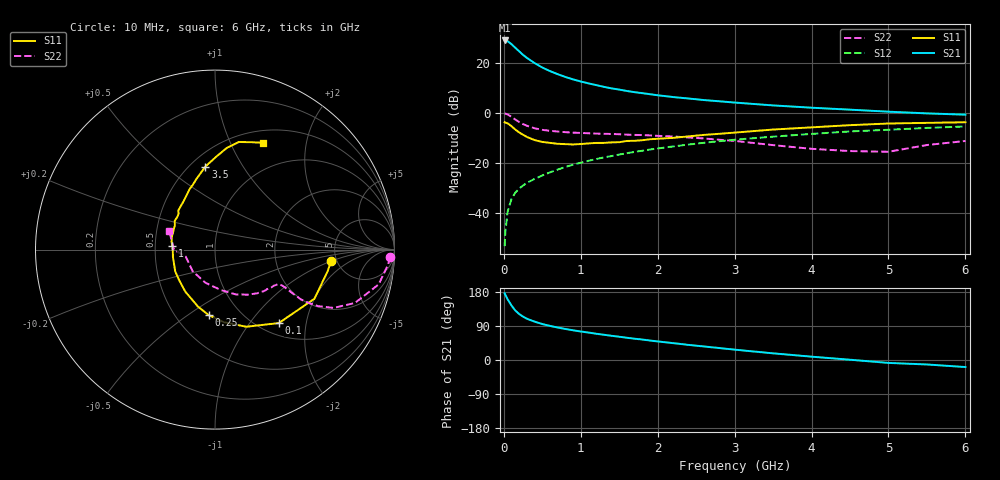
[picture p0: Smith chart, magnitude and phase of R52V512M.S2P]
! SIEMENS Small Signal Semiconductors
! BFR183
! Si NPN RF Bipolar Junction Transistor in SOT23
! VCE = 2.5 V  IC = 12 mA
! Common Emitter S-Parameters:  May  1996
# GHz  S  MA  R  50
!  f  S11  S21  S12  S22
! GHz  MAG  ANG  MAG  ANG  MAG  ANG  MAG  ANG
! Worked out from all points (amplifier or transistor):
!   36 points, 10 MHz to 6 GHz, reference 50 ohm
!   highest |S21| = 28.9 dB at 10 MHz (marker M1)
!   |S21| within 3 dB of that: start of sweep to 151.7 MHz
!   unconditionally stable (mu >= 1): 696 MHz to 2.461 GHz
!   at 250 MHz: K = 0.68, MSG = 26.1 dB, |S12| = -29.0 dB
!   at 1.4 GHz: K = 1.06, MAG = 12.1 dB, |S12| = -17.2 dB
!   at 6 GHz: K = 0.90, MSG = 2.3 dB, |S12| = -5.4 dB
!   S11 on the Smith chart (normalised r, x): 10 MHz: 4.49, -0.95; 100 MHz: 1.21, -1.41; 250 MHz: 0.72, -0.60; 1 GHz: 0.61, +0.03; 3.5 GHz: 0.59, +0.70; 6 GHz: 0.64, +1.33
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0.01  0.6494 -5.4  27.82 175.9  0.0022 84.9  0.9757 -2.4
0.02  0.6392 -10.9  27.72 171.6  0.0043 85.0  0.9686 -4.9
0.05  0.6178 -26.3  26.83 160.0  0.0109 80.0  0.9322 -12.0
0.1  0.5423 -49.0  23.42 143.6  0.0193 70.7  0.8341 -20.9
0.15  0.4639 -67.9  19.81 130.3  0.0259 66.9  0.736 -26.2
0.2  0.4076 -83.0  16.84 121.3  0.031 64.6  0.6558 -28.7
0.25  0.3663 -95.6  14.34 114.4  0.0356 63.6  0.5965 -29.7
0.3  0.3311 -106.7  12.49 108.9  0.0403 63.8  0.5535 -30.1
0.4  0.2871 -125.0  9.847 101.2  0.0483 64.9  0.494 -29.4
0.5  0.2634 -139.0  8.023 94.9  0.0564 66.1  0.459 -28.7
0.6  0.2526 -151.4  6.814 90.0  0.0652 66.3  0.4392 -28.3
0.7  0.2421 -160.4  5.914 85.6  0.0742 67.1  0.4247 -28.2
0.8  0.238 -170.1  5.204 81.9  0.0834 67.2  0.4127 -28.3
1  0.2392 174.9  4.227 75.2  0.1014 67.0  0.3982 -29.1
1.1  0.246 169.6  3.878 72.4  0.1108 66.7  0.3926 -30.2
1.3  0.2522 158.0  3.307 66.6  0.1294 65.7  0.3831 -32.0
1.6  0.2758 144.5  2.733 58.7  0.1573 63.4  0.3684 -36.1
2.2  0.3177 124.3  2.071 44.5  0.2143 58.1  0.3384 -46.0
3.5  0.4656 96.6  1.41 17.6  0.3362 42.7  0.2277 -81.8
4.5  0.5692 83.5  1.16 0.7  0.427 30.1  0.1733 -135.9
5.5  0.6327 71.0  0.978 -11.8  0.5014 18.2  0.2288 -179.9
6  0.6512 66.0  0.921 -18.6  0.5367 10.5  0.2754 157.9
